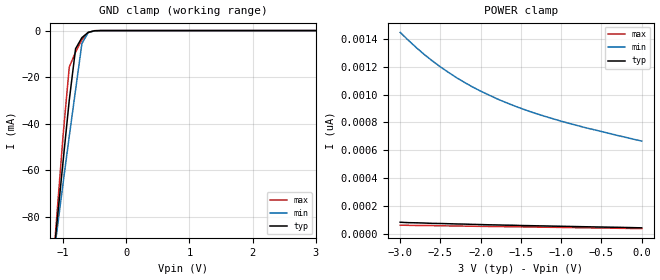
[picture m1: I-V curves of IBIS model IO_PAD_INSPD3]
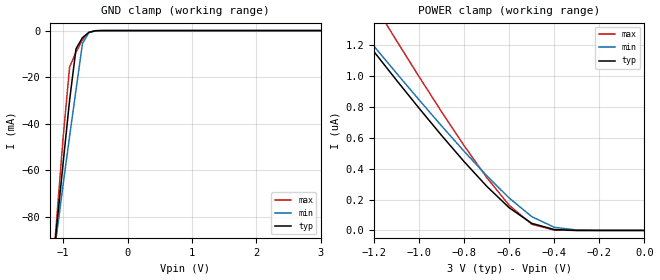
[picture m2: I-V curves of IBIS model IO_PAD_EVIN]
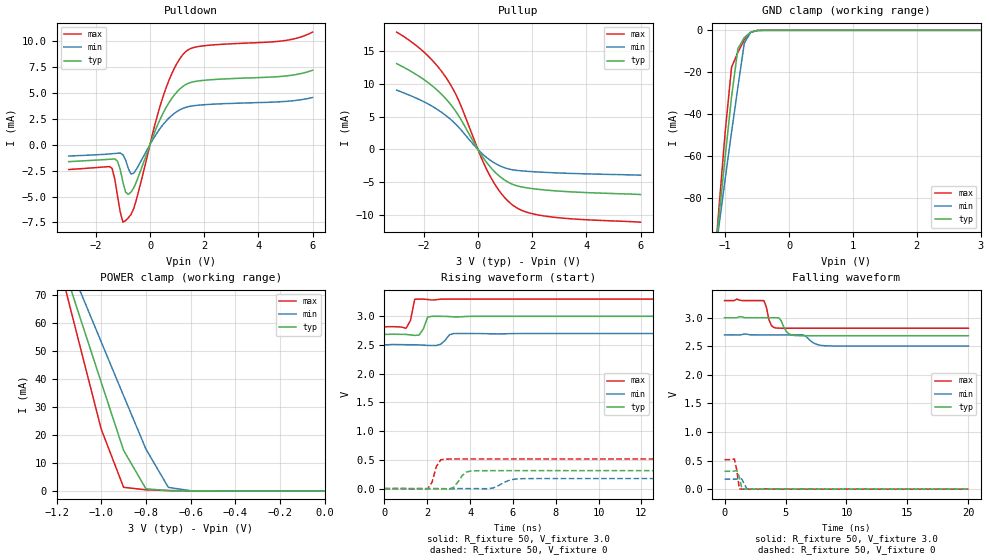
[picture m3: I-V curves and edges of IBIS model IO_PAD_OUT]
[IBIS Ver]   3.2
[Comment Char]   |_char
[File name]   r8804ce_30v.ibs
[File Rev]   1.0
[Date]   2018/09/06 11:25:17
[Source]
[Notes]
[Disclaimer]
This information is for modeling purposes only, and is not guaranteed.
Property of SEIKO EPSON Corp.,
unauthorized reproduction and/or distribution is strictly prohibited.
[Copyright]
Copyright 2018, SEIKO EPSON Corp.
[Component]   r8804ce50v
Si_location Pin
Timing_location Pin
[Manufacturer]   SEIKO EPSON Corp.
| RA/RX-8804CE
[Package]
R_pkg   267m   NA   NA
L_pkg   2.8nH   NA   NA
C_pkg   0.70pF   NA   NA
[Pin] signal_name   model_name
1   FOE   IO_PAD_INSPD3
2   Vdd   POWER
3   EVIN   IO_PAD_EVIN
4   FOUT   IO_PAD_OUT
5   SCL   IO_PAD_INSPD2
6   SOUT   IO_PAD_DIO
7   SDA   IO_PAD_DIO_SMT
8   Vpp   POWER
9   GND   GND
10   /INT   IO_PAD_XINT
| Models and submodels in the file (7): IO_PAD_INSPD3 (Input), IO_PAD_EVIN (Input), IO_PAD_OUT (3-state), IO_PAD_INSPD2 (Input), IO_PAD_DIO (I/O), IO_PAD_DIO_SMT (I/O_open_drain), IO_PAD_XINT (Open_drain)
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[Model]   IO_PAD_INSPD3
Model_type Input
Enable Active-High
Polarity Non-Inverting
Vinh=2.64
Vinl=0.54
C_comp   2.5p   2.0p   3.0p
[Temperature Range] 25   105   -40
[Voltage Range]   3.0   2.7   3.3
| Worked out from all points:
|   GND clamp passes 1 mA (typ) near -0.61 V on its own axis
[GND Clamp]
-3V       -618.7mA   -508.2mA   -765.2mA
-1.2V     -111.6mA   -108.8mA   -116mA
-1.1V     -84.12mA   -87.28mA   -80.81mA
-1V       -56.82mA   -66.05mA   -45.85mA
-900mV    -29.96mA   -45.45mA   -15.68mA
-800mV    -7.806mA   -25.47mA   -9.236mA
-700mV    -3.032mA   -5.588mA   -3.961mA
-600mV    -756.3uA   -818.4uA   -830.7uA
-500mV    -74.57uA   -117.4uA   -45.32uA
-400mV    -4.08uA    -12.66uA   -921.8nA
3V        45.59pA    707pA      35.81pA
[POWER Clamp]
-3V       85.72pA    1.445nA    64.8pA
-2.8V     81.63pA    1.336nA    62.53pA
-2.7V     80.04pA    1.286nA    62.76pA
-2.5V     76.62pA    1.198nA    60.03pA
-2.3V     73.33pA    1.121nA    58.66pA
-2.2V     72.42pA    1.086nA    57.98pA
-2V       69.12pA    1.024nA    56.27pA
-1.8V     66.51pA    970.1pA    54.8pA
-1.4V     61.39pA    880.7pA    51.5pA
-1V       56.96pA    809pA      48.66pA
-700mV    53.43pA    763pA      45.93pA
0V        45.59pA    666.7pA    39.79pA
[Model]   IO_PAD_EVIN
Model_type Input
Enable Active-High
Polarity Non-Inverting
Vinh=2.64
Vinl=0.54
C_comp   2.5p   2.0p   3.0p
[Temperature Range] 25   105   -40
[Voltage Range]   3.0   2.7   3.3
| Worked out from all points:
|   GND clamp passes 1 mA (typ) near -0.61 V on its own axis
[GND Clamp]
-3V       -618.7mA   -508.2mA   -765.2mA
-1.2V     -111.6mA   -108.8mA   -116mA
-1.1V     -84.12mA   -87.28mA   -80.81mA
-1V       -56.82mA   -66.05mA   -45.85mA
-900mV    -29.96mA   -45.45mA   -15.68mA
-800mV    -7.806mA   -25.47mA   -9.236mA
-700mV    -3.032mA   -5.588mA   -3.961mA
-600mV    -756.3uA   -818.4uA   -830.7uA
-500mV    -74.57uA   -117.4uA   -45.32uA
-400mV    -4.08uA    -12.66uA   -921.8nA
3V        45.59pA    2.885nA    34.9pA
[POWER Clamp]
-3V       4.792uA    4.57uA     6.082uA
-1.3V     1.346uA    1.371uA    1.708uA
-1.2V     1.158uA    1.194uA    1.467uA
-1.1V     973.3nA    1.019uA    1.23uA
-900mV    615.6nA    677.3nA    768.8nA
-800mV    445.9nA    512.8nA    549.4nA
-700mV    287nA      355.4nA    343.2nA
-600mV    147.3nA    210.2nA    163.3nA
-500mV    46.41nA    89.97nA    40.06nA
-400mV    5.98nA     20.52nA    2.649nA
-300mV    388.8pA    2.885nA    100.2pA
0V        45.59pA    666.6pA    39.79pA
[Model]   IO_PAD_OUT
Model_type 3-state
Enable Active-High
Polarity Non-Inverting
Vmeas=1.50
C_comp   2.5p   2.0p   3.0p
[Temperature Range] 25   105   -40
[Voltage Range]   3.0   2.7   3.3
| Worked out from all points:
|   slope of the pulldown table from 0 to 0.45 V, typ, clamps not added: 158 ohm
|   slope of the pullup table from 0 to 0.45 V, typ, clamps not added: 170 ohm
|   GND clamp passes 1 mA (typ) near -0.61 V on its own axis
|   POWER clamp passes 1 mA (typ) near -0.80 V on its own axis
|   falling waveform, R_fixture 50, V_fixture 3.0: 20-80 % time 461ps typ, 707ps min, 347ps max; typ from 3 V to 2.69 V
|   falling waveform, R_fixture 50, V_fixture 0: 20-80 % time 217ps typ, 254ps min, 227ps max; typ from 0.313 V to 0 V
|   rising waveform, R_fixture 50, V_fixture 3.0: 20-80 % time 216ps typ, 282ps min, 169ps max; typ from 2.69 V to 3 V
|   rising waveform, R_fixture 50, V_fixture 0: 20-80 % time 388ps typ, 569ps min, 261ps max; typ from 0 V to 0.313 V
[Pullup]
-3V       13.09mA    9.053mA    17.89mA
-2V       10.67mA    7.284mA    14.87mA
-1.6V     9.394mA    6.365mA    13.2mA
-1.2V     7.792mA    5.228mA    11.09mA
-700mV    5.066mA    3.34mA     7.375mA
100mV     -669uA     -419.1uA   -1.02mA
400mV     -2.398mA   -1.483mA   -3.684mA
800mV     -4.098mA   -2.481mA   -6.385mA
1.3V      -5.348mA   -3.117mA   -8.539mA
1.8V      -5.848mA   -3.325mA   -9.563mA
2.6V      -6.228mA   -3.518mA   -10.23mA
6V        -6.871mA   -3.923mA   -11.09mA
[Pulldown]
-3V       -1.645mA   -1.105mA   -2.404mA
-1.4V     -1.401mA   -881.9uA   -2.281mA
-1.2V     -1.594mA   -838.2uA   -4.933mA
-1V       -3.61mA    -971.9uA   -7.472mA
-800mV    -4.793mA   -2.307mA   -7.046mA
-600mV    -4.172mA   -2.75mA    -6.158mA
500mV     3.112mA    1.977mA    4.757mA
900mV     4.773mA    3.003mA    7.349mA
1.3V      5.744mA    3.563mA    8.902mA
2V        6.182mA    3.832mA    9.508mA
5V        6.596mA    4.15mA     10.01mA
6V        7.149mA    4.527mA    10.82mA
[GND Clamp]
-3V       -666mA     -547.8mA   -822.2mA
-1.2V     -119.5mA   -117.1mA   -123.7mA
-1.1V     -89.88mA   -93.83mA   -85.77mA
-1V       -60.41mA   -70.86mA   -48.66mA
-900mV    -31.76mA   -48.51mA   -17.63mA
-800mV    -8.707mA   -26.99mA   -10.46mA
-700mV    -3.454mA   -6.077mA   -4.512mA
-600mV    -868.8uA   -933.9uA   -956.3uA
-500mV    -86.23uA   -135.8uA   -52.66uA
-400mV    -4.725uA   -14.7uA    -1.074uA
3V        33.08pA    62.06nA    19.21pA
[POWER Clamp]
-3V       534.7mA    444mA      655.9mA
-1.2V     87.98mA    92.05mA    84.88mA
-1.1V     63.38mA    72.67mA    53.4mA
-1V       38.87mA    53.34mA    22.09mA
-900mV    14.53mA    34.09mA    1.297mA
-800mV    753.7uA    14.98mA    407.8uA
-700mV    112.9uA    1.273mA    132.2uA
-600mV    21.58uA    77.12uA    21.07uA
0V        33.08pA    754.7pA    24.78pA
[Falling Waveform]
R_fixture=50
V_fixture=3.0
V_fixture_min=2.7
V_fixture_max=3.3
0s        3V         2.7V       3.3V
3.232ns   3V         2.7V       3.299V
3.838ns   3V         2.7V       2.865V
4.242ns   3.001V     2.7V       2.82V
4.646ns   2.948V     2.7V       2.817V
5.253ns   2.721V     2.7V       2.817V
5.859ns   2.688V     2.7V       2.817V
6.465ns   2.685V     2.699V     2.816V
8.283ns   2.685V     2.509V     2.816V
20ns      2.685V     2.505V     2.816V
[Falling Waveform]
R_fixture=50
V_fixture=0
V_fixture_min=0
V_fixture_max=0
0s        312.9mV    175.1mV    516.2mV
606.1ps   311.1mV    174.2mV    514.5mV
808.1ps   317.1mV    173.8mV    530.4mV
1.01ns    327.2mV    177.3mV    325.4mV
1.212ns   212.6mV    185.3mV    5.852mV
1.414ns   10.74mV    177.5mV    80.63uV
1.818ns   44.29uV    10.16mV    1.427uV
2.02ns    927.2nV    1.763mV    -413.2nV
3.434ns   -4.055uV   -1.88uV    5.227mV
20ns      0V         0V         0V
[Rising Waveform]
R_fixture=50
V_fixture=3.0
V_fixture_min=2.7
V_fixture_max=3.3
0s        2.685V     2.505V     2.816V
1.01ns    2.684V     2.506V     2.792V
1.212ns   2.677V     2.505V     2.925V
1.414ns   2.667V     2.505V     3.296V
1.616ns   2.673V     2.502V     3.3V
2.02ns    2.988V     2.494V     3.293V
2.222ns   3V         2.491V     3.283V
2.626ns   3V         2.514V     3.298V
3.232ns   2.99V      2.699V     3.3V
20ns      3V         2.7V       3.3V
[Rising Waveform]
R_fixture=50
V_fixture=0
V_fixture_min=0
V_fixture_max=0
0s        0V         0V         0V
2.02ns    -9.656mV   108uV      -2.832mV
2.222ns   -21.08uV   77.83uV    110.5mV
2.424ns   19.01uV    -223uV     386.8mV
2.828ns   -1.158mV   -3.435mV   513.2mV
3.232ns   22.27mV    -1.447mV   515.6mV
3.838ns   289.5mV    14.58uV    516.1mV
4.242ns   310.6mV    -369uV     516.2mV
6.465ns   312.9mV    172.6mV    516.2mV
20ns      312.9mV    175.1mV    516.2mV
[Ramp]
R_load=50
dV/dt_r   1.877E-1/3.490E-10   1.051E-1/5.471E-10   3.097E-1/2.341E-10
dV/dt_f   1.891E-1/4.455E-10   1.172E-1/7.000E-10   2.901E-1/3.013E-10
|[End   IO_PAD_OUT
